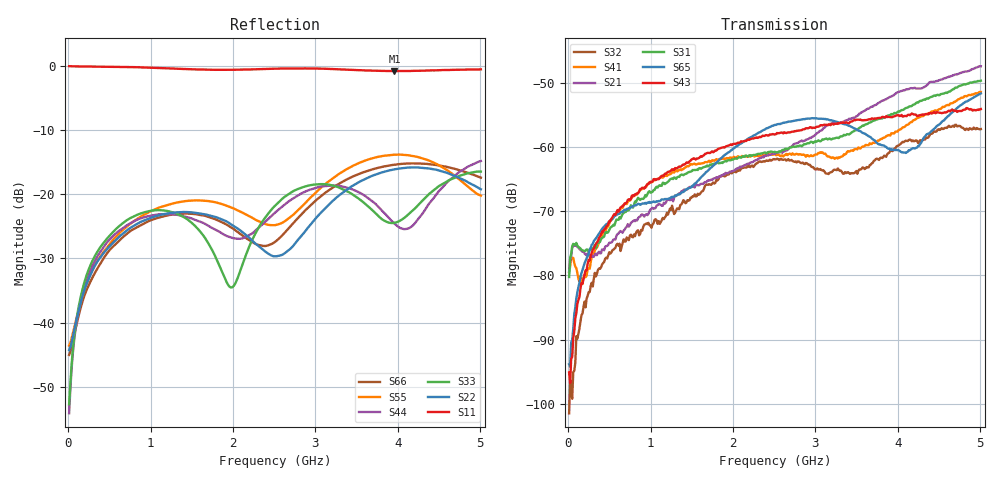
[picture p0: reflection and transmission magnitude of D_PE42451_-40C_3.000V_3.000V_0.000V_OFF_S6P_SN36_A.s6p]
! Device ID: PE42451
! Serial: 36
! Insertion: A
! Temp: -40C
! VDD: 3.000
! Control_Hi: 100.000
! Control_Lo: 0.000
! Logic State: OFF
! Port 1: RFC
! Port 2: RF1
! Port 3: RF2
! Port 4: RF3
! Port 5: RF4
! Port 6: RF5
! V1 = 0.00
! V2 = 3.00
! V3 = 3.00
! V4 = 0.00
! IDD: 1.312320e-05
#  Hz  S  RI  R  50
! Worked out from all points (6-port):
!   401 points, 10 MHz to 5.01 GHz, reference 50 ohm
!   strongest paths, dB at 10 MHz, 1.26 GHz, 2.51 GHz, 3.76 GHz, 5.01 GHz:
!     S43: -95.1, -63.5, -58.1, -55.5, -54.1
!     S65: -93.9, -67.8, -56.6, -59.5, -51.7
!     S31: -80.3, -64.9, -60.8, -55.7, -49.7
!     S21: -79.4, -68.0, -61.1, -53.2, -47.5
!     S41: -79.4, -63.9, -61.1, -59.0, -51.5
!     S32: -101.5, -69.2, -62.0, -61.9, -57.2
!   lowest |S11| = -0.9 dB at 3.96 GHz (marker M1), VSWR 19.91, Z = 2.75 - j15.3 ohm
!   |S11| at or under -10 dB: nowhere
